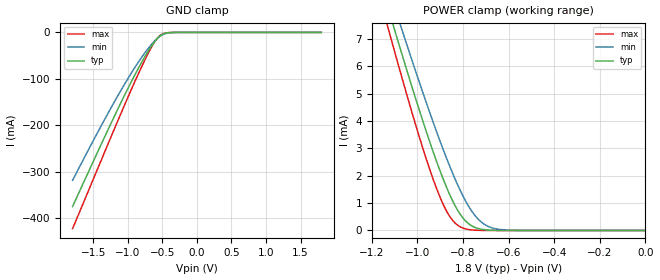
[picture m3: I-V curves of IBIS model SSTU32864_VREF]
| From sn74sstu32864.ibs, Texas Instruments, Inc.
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[Model]   SSTU32864_VREF
Model_type  Input
Vinl=0.844
Vinh=0.958
| variable   typ   min   max
C_comp   7.33pF   4.07pF   9.49pF
[Temperature Range]   40   85   0
| Ambient temperature   25   70   0
[Voltage range]   1.8   1.7   1.9
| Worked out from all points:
|   GND clamp passes 1 mA (typ) near -0.42 V on its own axis
|   POWER clamp passes 1 mA (typ) near -0.84 V on its own axis
[GND Clamp]
| SSTU32864_VREF
|   Voltage   I(typ)   I(min)   I(max)
-1.8V     -374.3mA   -318.1mA   -421.9mA
-1.34V    -226mA     -188.3mA   -258.6mA
-1V       -120.8mA   -99.54mA   -139.8mA
-830mV    -72.23mA   -60.02mA   -83.31mA
-690mV    -36.54mA   -31.66mA   -40.45mA
-605mV    -18.4mA    -17.38mA   -18.7mA
-535mV    -7.688mA   -8.402mA   -6.822mA
-450mV    -1.7mA     -2.357mA   -1.208mA
-310mV    -56.02uA   -146.1uA   -18.13uA
1.8V      5.386nA    29.89nA    2.269nA
[POWER Clamp]
| SSTU32864_VREF
|   Voltage   I(typ)   I(min)   I(max)
-1.8V     27.98mA    27.23mA    28.91mA
-1.135V   8.308mA    9.071mA    7.589mA
-1.12V    7.886mA    8.679mA    7.134mA
-1.095V   7.187mA    8.03mA     6.383mA
-1.065V   6.358mA    7.259mA    5.494mA
-975mV    3.964mA    5.006mA    2.968mA
-910mV    2.384mA    3.471mA    1.401mA
-860mV    1.337mA    2.381mA    534.5uA
-810mV    562.4uA    1.423mA    122.1uA
-735mV    74.96uA    425.3uA    6.79uA
-660mV    5.748uA    67.17uA    315.3nA
-16.28fV  5.386nA    28.43nA    2.461nA
